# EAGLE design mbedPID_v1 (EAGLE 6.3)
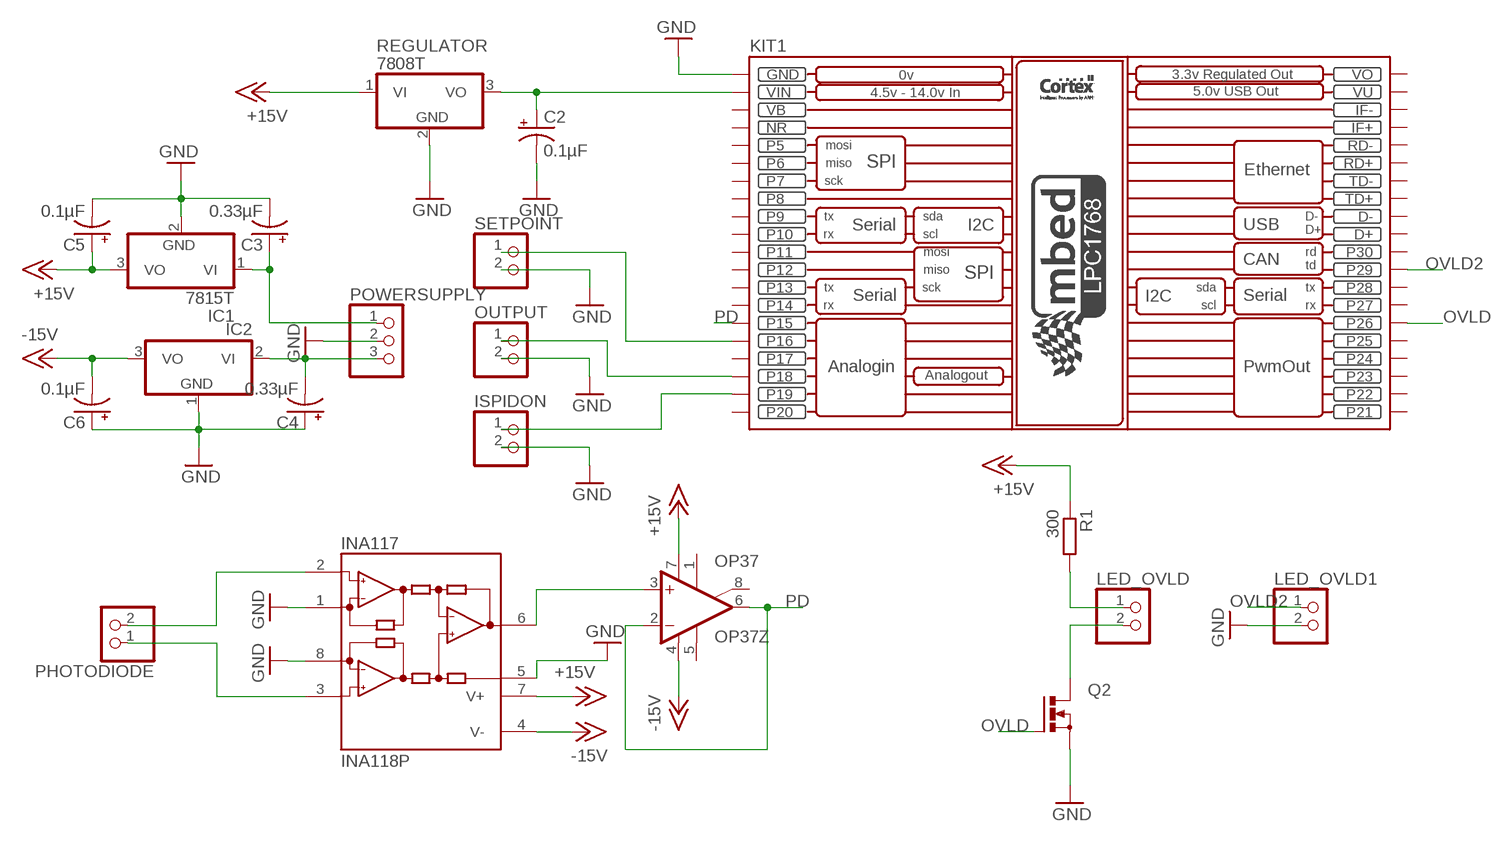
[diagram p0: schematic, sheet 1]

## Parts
C2  0.1µF  CPOL-USE2-5  [E2-5]
C3  0.33µF  CPOL-USE2-5  [E2-5]
C4  0.33µF  CPOL-USE2-5  [E2-5]
C5  0.1µF  CPOL-USE2-5  [E2-5]
C6  0.1µF  CPOL-USE2-5  [E2-5]
IC1  7815T  [TO220H]
IC2  7915T  [TO220H]
INA117  INA118P  [DIL08]
ISPIDON  PINHD-1X2  [1X02]
KIT1  MBED_NXP_LPC1768  [MBED-KIT]
LED_OVLD  PINHD-1X2  [1X02]
LED_OVLD1  PINHD-1X2  [1X02]
OP37  OP37Z  [DIL08]
OUTPUT  PINHD-1X2  [1X02]
PHOTODIODE  PINHD-1X2  [1X02]
POWERSUPPLY  PINHD-1X3  [1X03]
Q2  PMOSFET_NTO220BV  [TO220BV]
R1  300  R-EU_0207/10  [0207/10]
REGULATOR  7808T  [TO220H]
SETPOINT  PINHD-1X2  [1X02]

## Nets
+15V: C5.+ IC1.3(VO) INA117.7(V+) OP37.7(V+) R1.1 REGULATOR.1(VI)
-15V: C6.- IC2.3(VO) INA117.4(V-) OP37.4(V-)
GND: C2.- C3.- C4.+ C5.- C6.+ IC1.2(GND) IC2.1(GND) INA117.1(RG) INA117.5(REF) INA117.8(RG) ISPIDON.2 KIT1.GND LED_OVLD1.2 OUTPUT.2 POWERSUPPLY.2 Q2.S REGULATOR.2(GND) SETPOINT.2
N$1: C4.- IC2.2(VI) POWERSUPPLY.3
N$2: C3.+ IC1.1(VI) POWERSUPPLY.1
N$8: C2.+ KIT1.VIN REGULATOR.3(VO)
N$9: INA117.6(OUT) OP37.3(+IN)
N$10: KIT1.P$16(P16) SETPOINT.1
N$11: INA117.2(-IN) PHOTODIODE.2
N$12: KIT1.P$18(P18) OUTPUT.1
N$14: LED_OVLD.1 R1.2
N$15: LED_OVLD.2 Q2.D
N$16: ISPIDON.1 KIT1.P$19(P19)
OVLD: KIT1.P$26(P26) Q2.G
OVLD2: KIT1.P$29(P29) LED_OVLD1.1
PD: KIT1.P$15(P15) OP37.2(-IN) OP37.6(OUT)
PHOTODIODE: INA117.3(+IN) PHOTODIODE.1
Unconnected: KIT1.D+ KIT1.D- KIT1.IF+ KIT1.IF- KIT1.P$5(P5) KIT1.P$6(P6) KIT1.P$7(P7) KIT1.P$8(P8) KIT1.P$9(P9) KIT1.P$10(P10) KIT1.P$11(P11) KIT1.P$12(P12) KIT1.P$13(P13) KIT1.P$14(P14) KIT1.P$17(P17) KIT1.P$20(P20) KIT1.P$21(P21) KIT1.P$22(P22) KIT1.P$23(P23) KIT1.P$24(P24) KIT1.P$25(P25) KIT1.P$27(P27) KIT1.P$28(P28) KIT1.P$30(P30) KIT1.RD+ KIT1.RD- KIT1.TD+ KIT1.TD- OP37.1(ON1) OP37.5(OPT) OP37.8(ON2)

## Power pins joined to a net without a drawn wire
NR: KIT1.NR
VB: KIT1.VB
VO: KIT1.VOUT(VO)
VU: KIT1.VU

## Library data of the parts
C2-C6 = rcl:CPOL-US: POLARIZED CAPACITOR, American symbol
IC1 REGULATOR = linear:78*: Positive VOLTAGE REGULATOR Source: http://cache.national.com/ds/LM/LM78L05.pdf http://www.fairchildsemi.com/ds/LM/LM7805.pdf
IC2 = linear:79*: Negative VOLTAGE REGULATOR
INA117 = burr-brown:INA118: Instrumentation Amplifier Precision, Low Power; MF: TEXAS INSTRUMENTS; MPN: INA118P; OC_FARNELL: 1470354; OC_NEWARK: 96K4515
ISPIDON LED_OVLD LED_OVLD1 OUTPUT PHOTODIODE SETPOINT = pinhead:PINHD-1X2: PIN HEADER
KIT1 = MBED_v2.1:MBED_NXP_LPC1768: Mbed LPC1768 - ARM CORTEX v2.1 * Schematic symbol is now placed in eagles's default raster. *The pads diameter are suitable for routing between mbed pins * mbed pads are 0.8 mm drill diameter. --------------------------------------------- Created by: Mohamed Yousry *Alexandria, Egypt *Email: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
OP37 = linear:OP37: OP AMP
POWERSUPPLY = pinhead:PINHD-1X3: PIN HEADER
Q2 = transistor-power:PMOSFET_N: Power MOSFET N-Channel
R1 = rcl:R-EU_: RESISTOR, European symbol

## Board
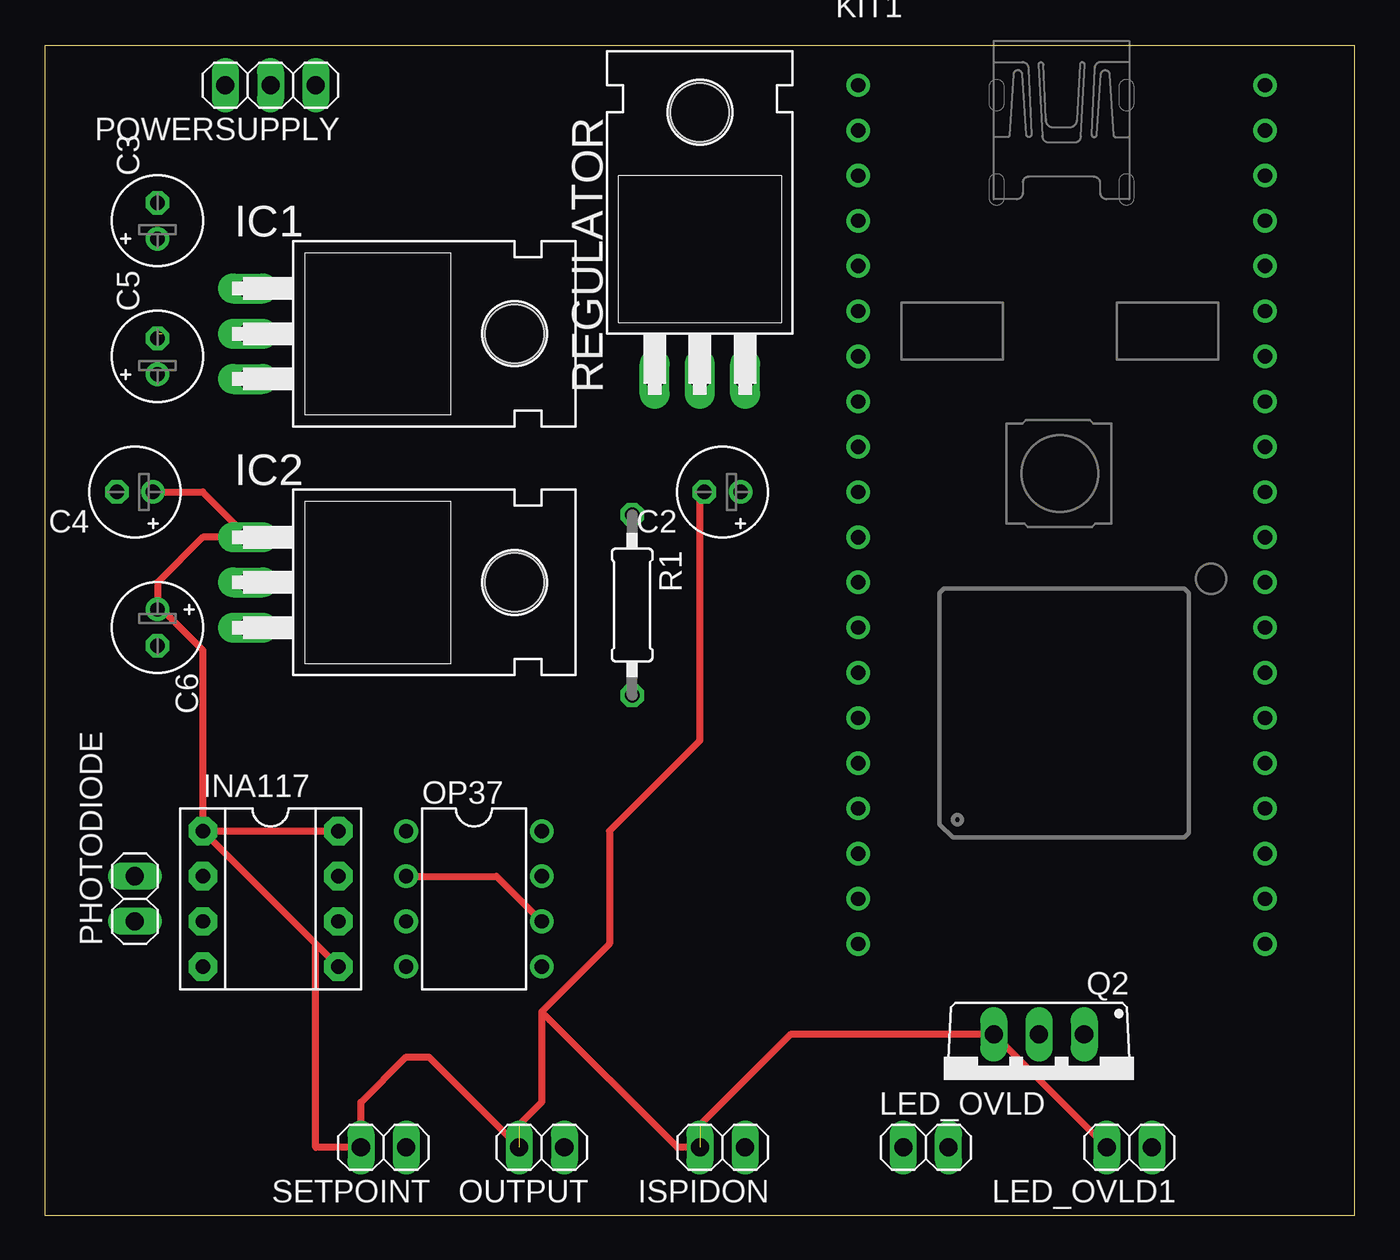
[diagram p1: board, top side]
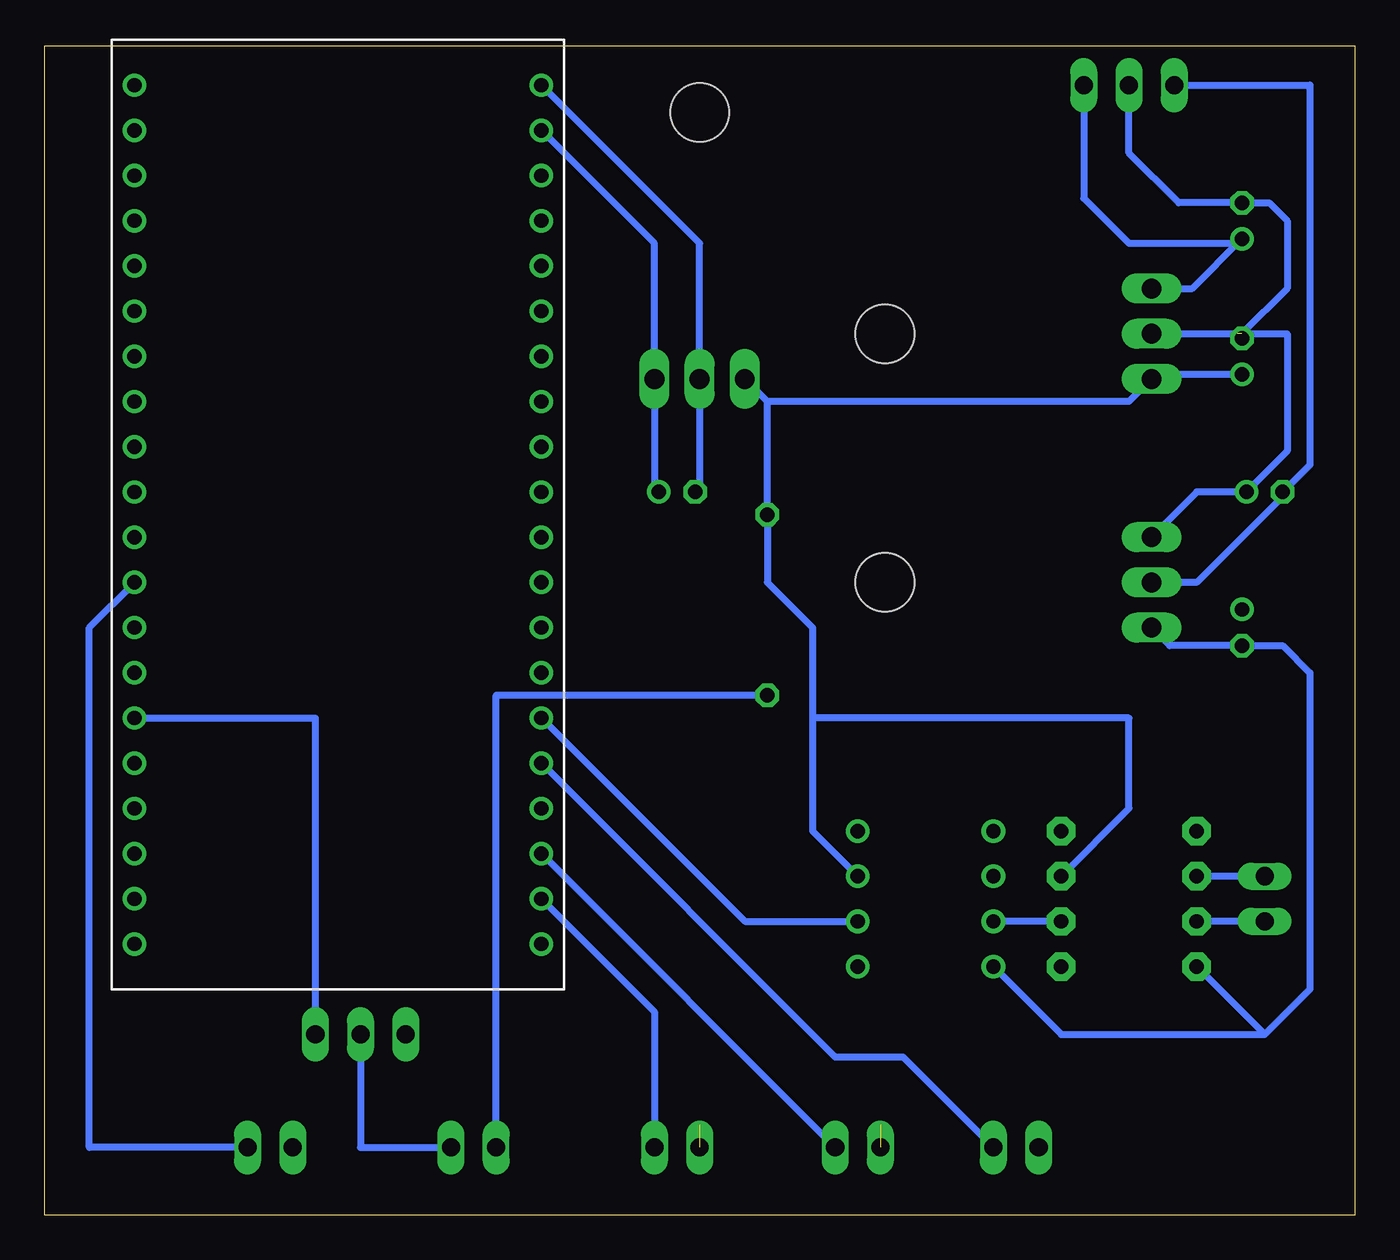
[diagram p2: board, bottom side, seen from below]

Size 73.64 x 65.71 mm. Coordinates in mm from the lower left corner, seen from the top.
Outline: 0,0 73.64,0 73.64,65.71 0,65.71 0,0
Copper layers (1*16): Top 0.035mm / dielectric 1.5mm / Bottom 0.035mm
Design rules "default": minimum track width 10mil, minimum drill 24mil, track to track 8mil, track to pad 8mil, pad to pad 8mil, via to via 8mil, smd to smd 8mil, copper to edge 40mil, drill to drill 8mil, minimum pad ring 10mil, minimum via ring 8mil, stop-mask expansion 4mil, vias tented up to drill 0mil, thermal gap 10mil

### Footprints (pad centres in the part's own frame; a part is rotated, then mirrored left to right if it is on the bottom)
E2-5 = drill 0.813 pad 1.27: + -1.016,0 | drill 0.813 pad 1.27 octagon: - 1.016,0
TO220H = drill 1.118 long: 1 -2.54,-10.16; 2 0,-10.16; 3 2.54,-10.16 | hole 3.302: 0,4.826
DIL08 = drill 0.813 pad 1.6 octagon: 1 -3.81,-3.81; 2 -1.27,-3.81; 3 1.27,-3.81; 4 3.81,-3.81; 5 3.81,3.81; 6 1.27,3.81; 7 -1.27,3.81; 8 -3.81,3.81
1X02 = drill 1.016 long: 1 -1.27,0; 2 1.27,0
MBED-KIT = drill 0.8: D+ 11.43,1.27; D- 11.43,3.81; GND -11.43,24.13; IF+ 11.43,16.51; IF- 11.43,19.05; NR -11.43,16.51; P$5 -11.43,13.97; P$6 -11.43,11.43; P$7 -11.43,8.89; P$8 -11.43,6.35; P$9 -11.43,3.81; P$10 -11.43,1.27; P$11 -11.43,-1.27; P$12 -11.43,-3.81; P$13 -11.43,-6.35; P$14 -11.43,-8.89; P$15 -11.43,-11.43; P$16 -11.43,-13.97; P$17 -11.43,-16.51; P$18 -11.43,-19.05; P$19 -11.43,-21.59; P$20 -11.43,-24.13; P$21 11.43,-24.13; P$22 11.43,-21.59; P$23 11.43,-19.05; P$24 11.43,-16.51; P$25 11.43,-13.97; P$26 11.43,-11.43; P$27 11.43,-8.89; P$28 11.43,-6.35; P$29 11.43,-3.81; P$30 11.43,-1.27; RD+ 11.43,11.43; RD- 11.43,13.97; TD+ 11.43,6.35; TD- 11.43,8.89; VB -11.43,19.05; VIN -11.43,21.59; VOUT 11.43,24.13; VU 11.43,21.59
DIL08' = drill 0.813 pad 1.27: 1 -3.81,-3.81; 2 -1.27,-3.81; 3 1.27,-3.81; 4 3.81,-3.81; 5 3.81,3.81; 6 1.27,3.81; 7 -1.27,3.81; 8 -3.81,3.81
1X03 = drill 1.016 long: 1 -2.54,0; 2 0,0; 3 2.54,0
TO220BV = drill 1.016 long: D 0,-2.54; G -2.54,-2.54; S 2.54,-2.54
0207/10 = drill 0.813 octagon: 1 -5.08,0; 2 5.08,0

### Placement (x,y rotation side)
C2  38.1,40.64 180 top
C3  6.35,55.88 90 top
C4  5.08,40.64 180 top
C5  6.35,48.26 90 top
C6  6.35,33.02 270 top
IC1  21.59,49.53 270 top
IC2  21.59,35.56 270 top
INA117  12.7,17.78 270 top
ISPIDON  38.1,3.81 180 top
KIT1  57.15,39.37 0 top
LED_OVLD  49.53,3.81 0 top
LED_OVLD1  60.96,3.81 180 top
OP37  OP37Z  [DIL08']  24.13,17.78 270 top
OUTPUT  27.94,3.81 180 top
PHOTODIODE  5.08,17.78 90 top
POWERSUPPLY  12.7,63.5 180 top
Q2  55.88,7.62 180 top
R1  33.02,34.29 270 top
REGULATOR  36.83,57.15 0 top
SETPOINT  19.05,3.81 180 top

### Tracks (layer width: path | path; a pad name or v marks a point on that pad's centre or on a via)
+15V
  Bottom 0.406: C5.+ 11.18,47.24 IC1.3 12.7,45.72 33.02,45.72 | 33.02,45.72 REGULATOR.1 | 33.02,45.72 R1.1 33.02,35.56 30.48,33.02 30.48,27.94 | 30.48,27.94 30.48,21.59 OP37.7 | INA117.7 12.7,22.86 12.7,27.94 30.48,27.94
-15V
  Bottom 0.406: IC2.3 10.41,32 C6.- 4.06,32 2.54,30.48 2.54,12.7 5.08,10.16 | OP37.4 16.51,10.16 5.08,10.16 | INA117.4 5.08,10.16
GND  (3 unrouted)
  Top 0.406: C4.+ 8.89,40.64 IC2.1 8.89,38.1 6.35,35.56 C6.+ 6.6,34.04 8.89,31.75 INA117.1 | INA117.1 INA117.8 | INA117.5 15.24,15.24 | 27.94,11.43 27.94,6.35 26.67,5.08 | ISPIDON.2 35.56,3.81 27.94,11.43 | 36.83,5.08 41.91,10.16 Q2.S LED_OVLD1.2 | C2.- 36.83,40.39 36.83,26.67 31.75,21.59 31.75,15.24 27.94,11.43 | 15.24,15.24 15.24,3.81 SETPOINT.2 17.78,6.35 20.32,8.89 21.59,8.89 OUTPUT.2 | 15.24,15.24 INA117.1
  Bottom 0.406: IC1.2 6.6,49.53 C5.- | POWERSUPPLY.2 12.7,59.69 9.91,56.9 C3.- 4.83,56.9 3.81,55.88 3.81,52.07 6.35,49.53 3.81,49.53 3.81,42.93 C4.+ 8.89,40.64 IC2.1 | C2.- 36.83,40.89 REGULATOR.2 36.83,54.61 KIT1.GND
N$1
  Bottom 0.406: POWERSUPPLY.3 2.54,63.5 2.54,42.16 C4.- 4.06,40.39 8.89,35.56 IC2.2
N$2
  Bottom 0.406: IC1.1 9.14,52.07 C3.+ 6.6,54.61 12.7,54.61 15.24,57.15 POWERSUPPLY.1
N$8
  Bottom 0.406: C2.+ 39.37,40.89 REGULATOR.3 39.37,54.61 KIT1.VIN
N$9
  Bottom 0.406: INA117.6 OP37.3
N$10
  Bottom 0.406: KIT1.P$16 29.21,8.89 25.4,8.89 SETPOINT.1
N$11
  Bottom 0.406: PHOTODIODE.2 INA117.2
N$12
  Bottom 0.406: KIT1.P$18 OUTPUT.1
N$14
  Bottom 0.406: R1.2 48.26,29.21 LED_OVLD.1
N$15
  Bottom 0.406: Q2.D 55.88,3.81 LED_OVLD.2
N$16
  Bottom 0.406: KIT1.P$19 39.37,11.43 ISPIDON.1
OVLD
  Bottom 0.406: KIT1.P$26 58.42,27.94 Q2.G
OVLD2
  Bottom 0.406: LED_OVLD1.1 71.12,3.81 71.12,33.02 KIT1.P$29
PD
  Top 0.406: OP37.2 25.4,19.05 OP37.6
  Bottom 0.406: KIT1.P$15 34.29,16.51 OP37.6
PHOTODIODE
  Bottom 0.406: PHOTODIODE.1 INA117.3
